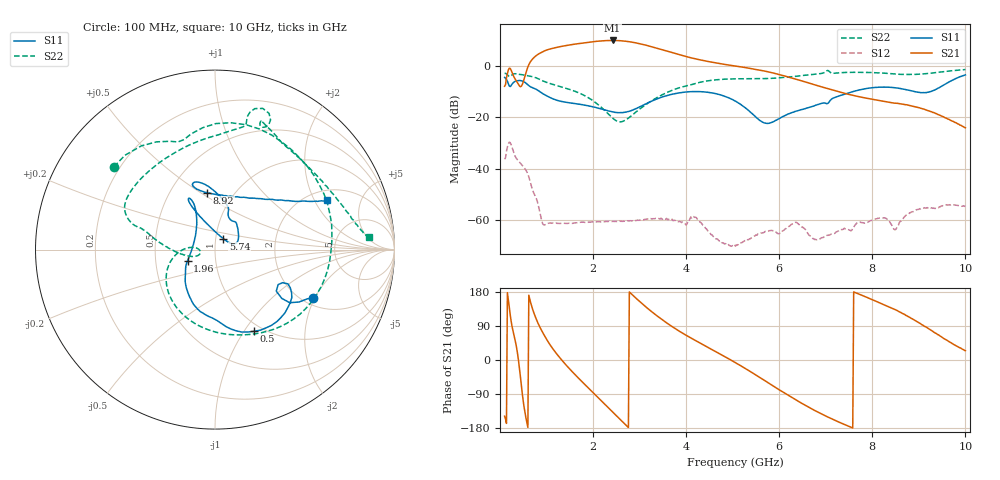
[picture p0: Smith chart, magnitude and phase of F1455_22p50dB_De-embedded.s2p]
! Integrated Device Technology
! Corporate Headquarters
! 6024 Silver Creek Valley Road
! San Jose, CA 95138  USA
! Phone:  1-408-284-8200
! Toll Free:  1-800-223-1366
! Webpage:  http://www.idt.com/
! Timing and RF Division
! 515 Groton Road, Suite 102
! Westford, MA 01886-6024
! Device:  F1455
! Description: 6-bit 0.5 dB Transmit Variable Gain Amplifier
! Frequency:  1400.0 -  2300.00 MHz
! Package:  6x6 mm Thin QFN Plastic Package: 28 pin
! State:  45
! Atten State:  22.5 dB
! Voltage:  +5.00 Volts
! Current:  217.612 mA
! Data:  The device was measured on a the F1455 evaluation board which has
!  individual transmission lines to the RF pins.  Data was collected
!  using a calibrated network analyzer.  The evaluation board was
!  de-embedded using a TRL calibration technique.
!  The reference plane is the edge of the package pin.
!  Pin  1 = CSb
!  Pin  2 = DATA
!  Pin  3 = CLK
!  Pin  4 = RSET
!  Pin  5 = GND
!  Pin  6 = RFIN  = Port 1
!  Pin  7 = GND
!  Pin  8 = NC
!  Pin  9 = NC
!  Pin 10 = NC
!  Pin 11 = NC
!  Pin 12 = NC
!  Pin 13 = NC
!  Pin 14 = /STBY
!  Pin 15 = GND
!  Pin 16 = RFOUT  = Port 2
!  Pin 17 = GND
!  Pin 18 = NC
!  Pin 19 = NC
!  Pin 20 = NC
!  Pin 21 = GND
!  Pin 22 = NC
!  Pin 23 = GND
!  Pin 24 = NC
!  Pin 25 = NC
!  Pin 26 = NC
!  Pin 27 = GND
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# GHz S dB R 50
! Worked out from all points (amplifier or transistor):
!   496 points, 100 MHz to 10 GHz, reference 50 ohm
!   highest |S21| = 10.1 dB at 2.42 GHz (marker M1)
!   |S21| within 3 dB of that: 1.15 GHz to 3.371 GHz (2.221 GHz wide, 98.2 % of centre)
!   unconditionally stable (mu >= 1): start of sweep to end of sweep
!   at 1.74 GHz: K = 175.65, MAG = 9.6 dB, |S12| = -61.0 dB
!   at 5.06 GHz: K = 1055.36, MAG = 2.0 dB, |S12| = -70.4 dB
!   at 10 GHz: K = 599.89, MAG = -15.4 dB, |S12| = -54.8 dB
!   S11 on the Smith chart (normalised r, x): 100 MHz: 2.27, -1.93; 500 MHz: 0.91, -1.11; 1.96 GHz: 0.73, -0.09; 5.74 GHz: 1.09, +0.13; 8.92 GHz: 0.76, +0.53; 10 GHz: 2.46, +2.52
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0.1  -4.32 -26.1  -7.79 -148.4  -36.37 46.9  -2.76 140.7
0.18  -6.73 -36.2  -1.44 159.9  -30.29 -6.9  -3.69 112.7
0.26  -6.94 -25.1  -2.40 88.3  -31.77 -76.7  -3.32 95.9
0.38  -5.59 -42.3  -6.52 15.2  -36.69 -117.6  -3.03 58.0
0.5  -5.93 -64.4  -6.10 -108.3  -39.21 -156.3  -3.33 26.9
0.68  -8.22 -90.4  2.44 142.6  -47.15 137.5  -3.98 -14.7
0.82  -9.46 -108.8  4.71 96.5  -54.05 107.9  -4.83 -45.7
0.96  -11.11 -123.5  6.07 63.4  -62.09 126.4  -5.99 -71.1
1.34  -13.79 -143.6  7.87 -2.0  -61.45 103.5  -8.15 -121.6
1.76  -14.98 -153.4  9.09 -56.9  -61.02 71.9  -10.92 -158.3
1.96  -15.70 -158.1  9.56 -81.1  -60.93 62.2  -12.98 -171.8
2.42  -17.79 179.3  10.12 -137.0  -60.69 44.6  -20.27 176.5
2.82  -17.34 142.4  9.51 174.8  -60.46 33.9  -19.41 -161.1
3.1  -14.99 124.9  8.43 143.7  -59.96 28.2  -15.44 -169.7
3.4  -12.56 116.8  6.97 114.2  -59.51 16.6  -11.99 178.8
4.08  -9.93 116.3  3.44 59.7  -59.70 4.6  -7.32 163.8
5.06  -13.63 114.8  0.10 -7.0  -70.38 7.6  -4.89 148.5
5.74  -22.35 52.8  -2.06 -58.3  -64.61 15.3  -4.78 120.2
6.7  -15.78 37.3  -6.88 -129.1  -66.81 -136.6  -3.21 78.6
8.36  -8.19 108.4  -14.07 139.8  -60.49 78.3  -2.82 62.5
8.92  -9.92 97.7  -15.85 104.3  -56.42 102.2  -3.15 40.0
10  -3.34 23.9  -24.07 24.7  -54.76 29.1  -1.28 4.6
